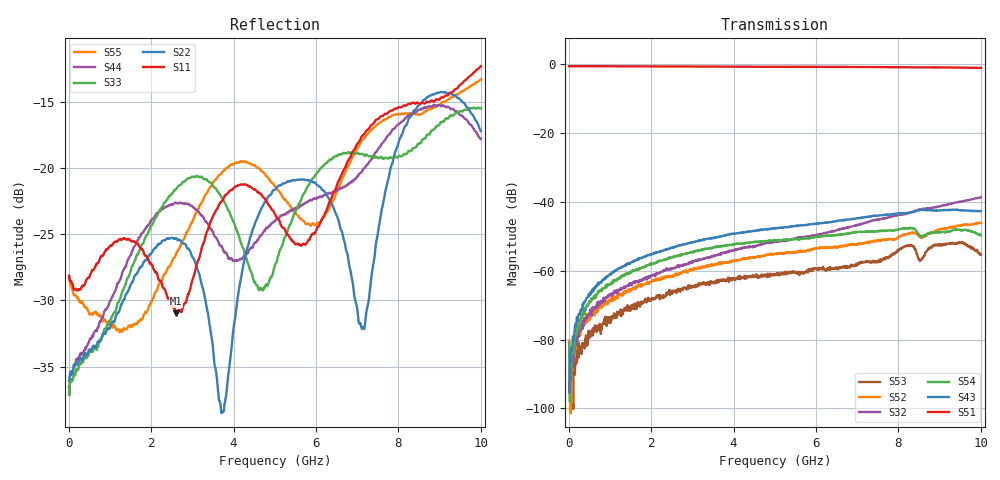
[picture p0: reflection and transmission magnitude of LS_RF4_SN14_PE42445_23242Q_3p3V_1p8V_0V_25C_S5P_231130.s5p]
!Keysight Technologies,M9804A,MY58100185,A.15.10.06
!Date: Thursday, November 30, 2023 12:05:19
!Correction: S11(Cdelta 6-Port  )
!S12(Cdelta 6-Port  )
!S13(Cdelta 6-Port  )
!S15(Cdelta 6-Port  )
!S16(Cdelta 6-Port  )
!S21(Cdelta 6-Port  )
!S22(Cdelta 6-Port  )
!S23(Cdelta 6-Port  )
!S25(Cdelta 6-Port  )
!S26(Cdelta 6-Port  )
!S31(Cdelta 6-Port  )
!S32(Cdelta 6-Port  )
!S33(Cdelta 6-Port  )
!S35(Cdelta 6-Port  )
!S36(Cdelta 6-Port  )
!S51(Cdelta 6-Port  )
!S52(Cdelta 6-Port  )
!S53(Cdelta 6-Port  )
!S55(Cdelta 6-Port  )
!S56(Cdelta 6-Port  )
!S61(Cdelta 6-Port  )
!S62(Cdelta 6-Port  )
!S63(Cdelta 6-Port  )
!S65(Cdelta 6-Port  )
!S66(Cdelta 6-Port  )
!S5P File: Measurements: <S11,S12,S13,S15,S16>,
!<S21,S22,S23,S25,S26>,
!<S31,S32,S33,S35,S36>,
!<S51,S52,S53,S55,S56>,
!<S61,S62,S63,S65,S66>:
# Hz S  dB  R 50
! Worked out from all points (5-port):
!   1000 points, 10 MHz to 10 GHz, reference 50 ohm
!   strongest paths, dB at 10 MHz, 2.51 GHz, 5.01 GHz, 7.51 GHz, 10 GHz:
!     S51: -0.6, -0.6, -0.7, -0.8, -1.0
!     S43: -92.3, -53.3, -47.6, -44.0, -42.7
!     S54: -81.0, -56.1, -51.1, -48.4, -49.7
!     S32: -91.6, -59.4, -51.6, -45.1, -38.7
!     S52: -80.3, -61.6, -55.1, -51.2, -46.1
!     S53: -80.9, -66.7, -61.0, -57.1, -55.2
!   lowest |S11| = -31.0 dB at 2.61 GHz (marker M1), VSWR 1.06, Z = 50.8 - j2.74 ohm
!   |S11| at or under -10 dB: start of sweep to end of sweep
